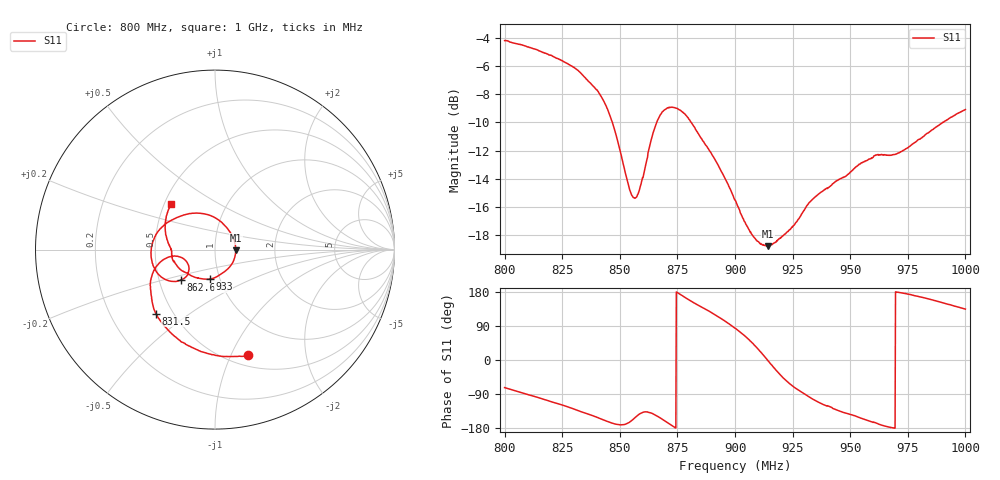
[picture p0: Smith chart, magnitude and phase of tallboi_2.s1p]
# HZ S RI R 50
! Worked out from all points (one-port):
!   1010 points, 800 MHz to 1 GHz, reference 50 ohm
!   lowest |S11| = -18.8 dB at 914.4 MHz (marker M1), VSWR 1.26, Z = 63 - j0.587 ohm
!   |S11| at or under -10 dB: 846.8 MHz to 866 MHz (19.26 MHz wide, 2.25 % of centre); 881 MHz to 990.2 MHz (109.2 MHz wide, 11.7 % of centre)
!   S11 on the Smith chart (normalised r, x): 800 MHz: 0.61, -1.16; 831.5 MHz: 0.40, -0.38; 862.6 MHz: 0.65, -0.24; 933 MHz: 0.89, -0.30; 1 GHz: 0.54, +0.31
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8e8  0.1823 -0.5894
8.132805e8  -0.069 -0.5701
8.251734e8  -0.2542 -0.4562
8.315163e8  -0.3292 -0.3571
8.416254e8  -0.3562 -0.1666
8.459861e8  -0.3185 -0.085
8.501486e8  -0.2475 -0.039
8.543112e8  -0.1749 -0.051
8.564916e8  -0.1511 -0.0784
8.590684e8  -0.1463 -0.1201
8.626363e8  -0.1898 -0.1698
8.654113e8  -0.2517 -0.1745
8.681863e8  -0.3109 -0.1423
8.71556e8  -0.3502 -0.0697
8.751239e8  -0.3537 0.0166
8.810703e8  -0.2858 0.1338
8.868186e8  -0.1889 0.1879
8.933597e8  -0.0806 0.202
9.000991e8  0.0184 0.1666
9.076313e8  0.09 0.0878
9.143706e8  0.115 -0.0046
9.250743e8  0.048 -0.1268
9.330029e8  -0.0301 -0.1641
9.500495e8  -0.1696 -0.1253
9.613478e8  -0.2358 -0.0563
9.750247e8  -0.2556 0.0269
9.88107e8  -0.2779 0.1314
9.999999e8  -0.2453 0.2513
